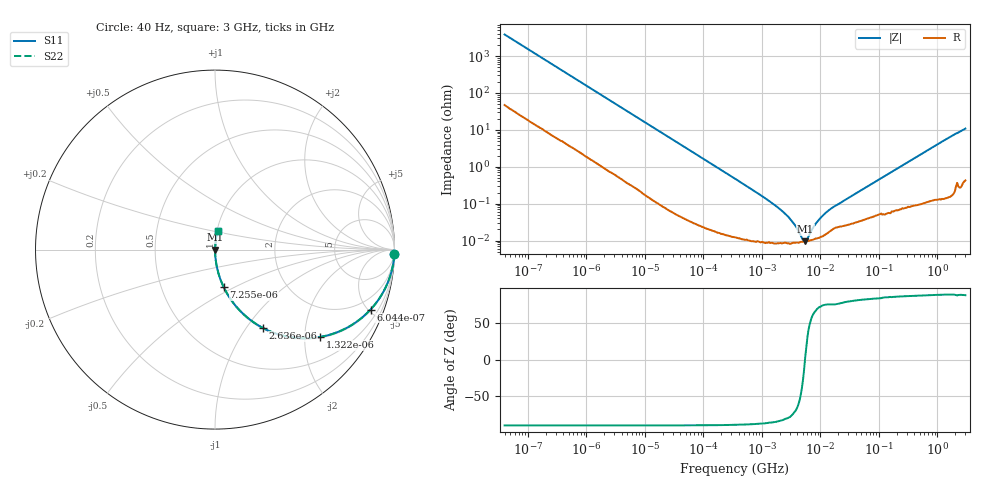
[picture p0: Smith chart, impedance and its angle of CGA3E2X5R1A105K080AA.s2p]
! S-parameter Generated by TDK Corporation
! Copyright(C) 2015 TDK Corporation.
! All Rights Reserved.
! TDK P/N: CGA3E2X5R1A105K080AA (Multilayer Ceramic Chip Capacitors)
! Property: C=1uF
! Size(LxWxT): 1.6x0.8x0.8mm, 0.063x0.031x0.031inches
! Model Type: s2p (Touchstone File Format Version 1.0)
! Frequency: DC=Yes Start=0.00004MHz Stop=3000MHz 396points Log-sweep
! Note: This model was converted from impedance.
! Model Generated on Jun. 23, 2015
! Hash(MD5):
! Port Assignments:
!  1 ---| |--- 2
! Applicable Conditions:
!  Temperature = 25 degC
!  DC Bias Voltage = 0 V
!  Small Signal Operation
! Terms and conditions regarding TDK Simulation Models
! (1)This simulation model is being provided solely for informational purposes. Please refer to the specifications of the products in terms of detailed characteristics of such products.
! (2)In no event shall TDK Corporation of any of its subsidiaries be liable for any loss or damage arising, directly or indirectly,
!  From any information contained in this simulation model, including, but not limited to loss or damages arising from any inaccuracies, omissions or errors in connection with such information.
! (3)Any and all copyrights on this simulation model are owned by TDK Corporation.
!  Duplication or redistribution of this simulation model without prior written permission from TDK Corporation is prohibited.
! (4)This simulation model is subject to any modification or change without any prior notice.
! (5)Neither TDK Corporation nor any of its subsidiaries shall make any warranty, express or implied,
!  Including but not limited to the correctness, implied warranties of merchantability and fitness for a particular purpose with respect to this simulation models.
! (6)The use of this simulation model shall be deemed to have consented to the terms and conditions hereof.
# MHz S MA R 50
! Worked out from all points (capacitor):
!   395 points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, 40 Hz to 3 GHz, reference 50 ohm
!   read as one part in series: C = 1.03 uF near 41.88 Hz
!   lowest |Z| = 9.61 mohm at 5.481 MHz (marker M1)
!   series resonance near 5.442 MHz, so ESL is about 830 pH
!   S11 on the Smith chart (normalised r, x): 40 Hz: 2, -77; 604.4 Hz: 1.06, -5.17; 1.322 kHz: 1.03, -2.37; 2.636 kHz: 1.01, -1.20; 7.255 kHz: 1.00, -0.44; 3 GHz: 1.01, +0.22
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4e-05  0.9993 -1.5  0.02599 87.8  0.02599 87.8  0.9993 -1.5
0.0001826612  0.9918 -6.7  0.1168 82.6  0.1168 82.6  0.9918 -6.7
0.0006043944  0.9288 -21.1  0.3595 68.2  0.3595 68.2  0.9288 -21.1
0.000834128  0.878 -27.9  0.4682 61.4  0.4682 61.4  0.878 -27.9
0.001321622  0.7604 -39.8  0.6405 49.5  0.6405 49.5  0.7604 -39.8
0.002635842  0.5106 -58.6  0.8539 30.7  0.8539 30.7  0.5106 -58.6
0.004176322  0.3532 -68.7  0.9315 20.7  0.9315 20.7  0.3532 -68.7
0.007255102  0.2139 -77.0  0.9744 12.4  0.9744 12.4  0.2139 -77.0
0.01739424  0.09208 -84.1  0.9948 5.3  0.9948 5.3  0.09208 -84.1
0.3464102  0.004752 -88.3  0.9999 0.3  0.9999 0.3  0.004752 -88.3
2.084979  0.0006873 -82.8  0.9999 0.0  0.9999 0.0  0.0006873 -82.8
3.303516  0.0003277 -74.9  0.9999 0.0  0.9999 0.0  0.0003277 -74.9
3.971241  0.0002149 -65.7  0.9999 0.0  0.9999 0.0  0.0002149 -65.7
4.998775  0.0001062 -29.3  0.9999 0.0  0.9999 0.0  0.0001062 -29.3
5.480732  9.614e-05 2.8  0.9999 -0.0  0.9999 -0.0  9.614e-05 2.8
5.738865  0.0001011 17.6  0.9999 -0.0  0.9999 -0.0  0.0001011 17.6
7.22376  0.0002024 59.1  0.9999 -0.0  0.9999 -0.0  0.0002024 59.1
9.969551  0.0004063 72.1  0.9999 -0.0  0.9999 -0.0  0.0004063 72.1
15.08561  0.0007307 75.3  0.9998 -0.0  0.9998 -0.0  0.0007307 75.3
150.6385  0.006631 84.8  0.9994 -0.4  0.9994 -0.4  0.006631 84.8
865.884  0.03541 86.0  0.9981 -2.0  0.9981 -2.0  0.03541 86.0
3000  0.1072 81.6  0.99 -6.1  0.99 -6.1  0.1072 81.6
